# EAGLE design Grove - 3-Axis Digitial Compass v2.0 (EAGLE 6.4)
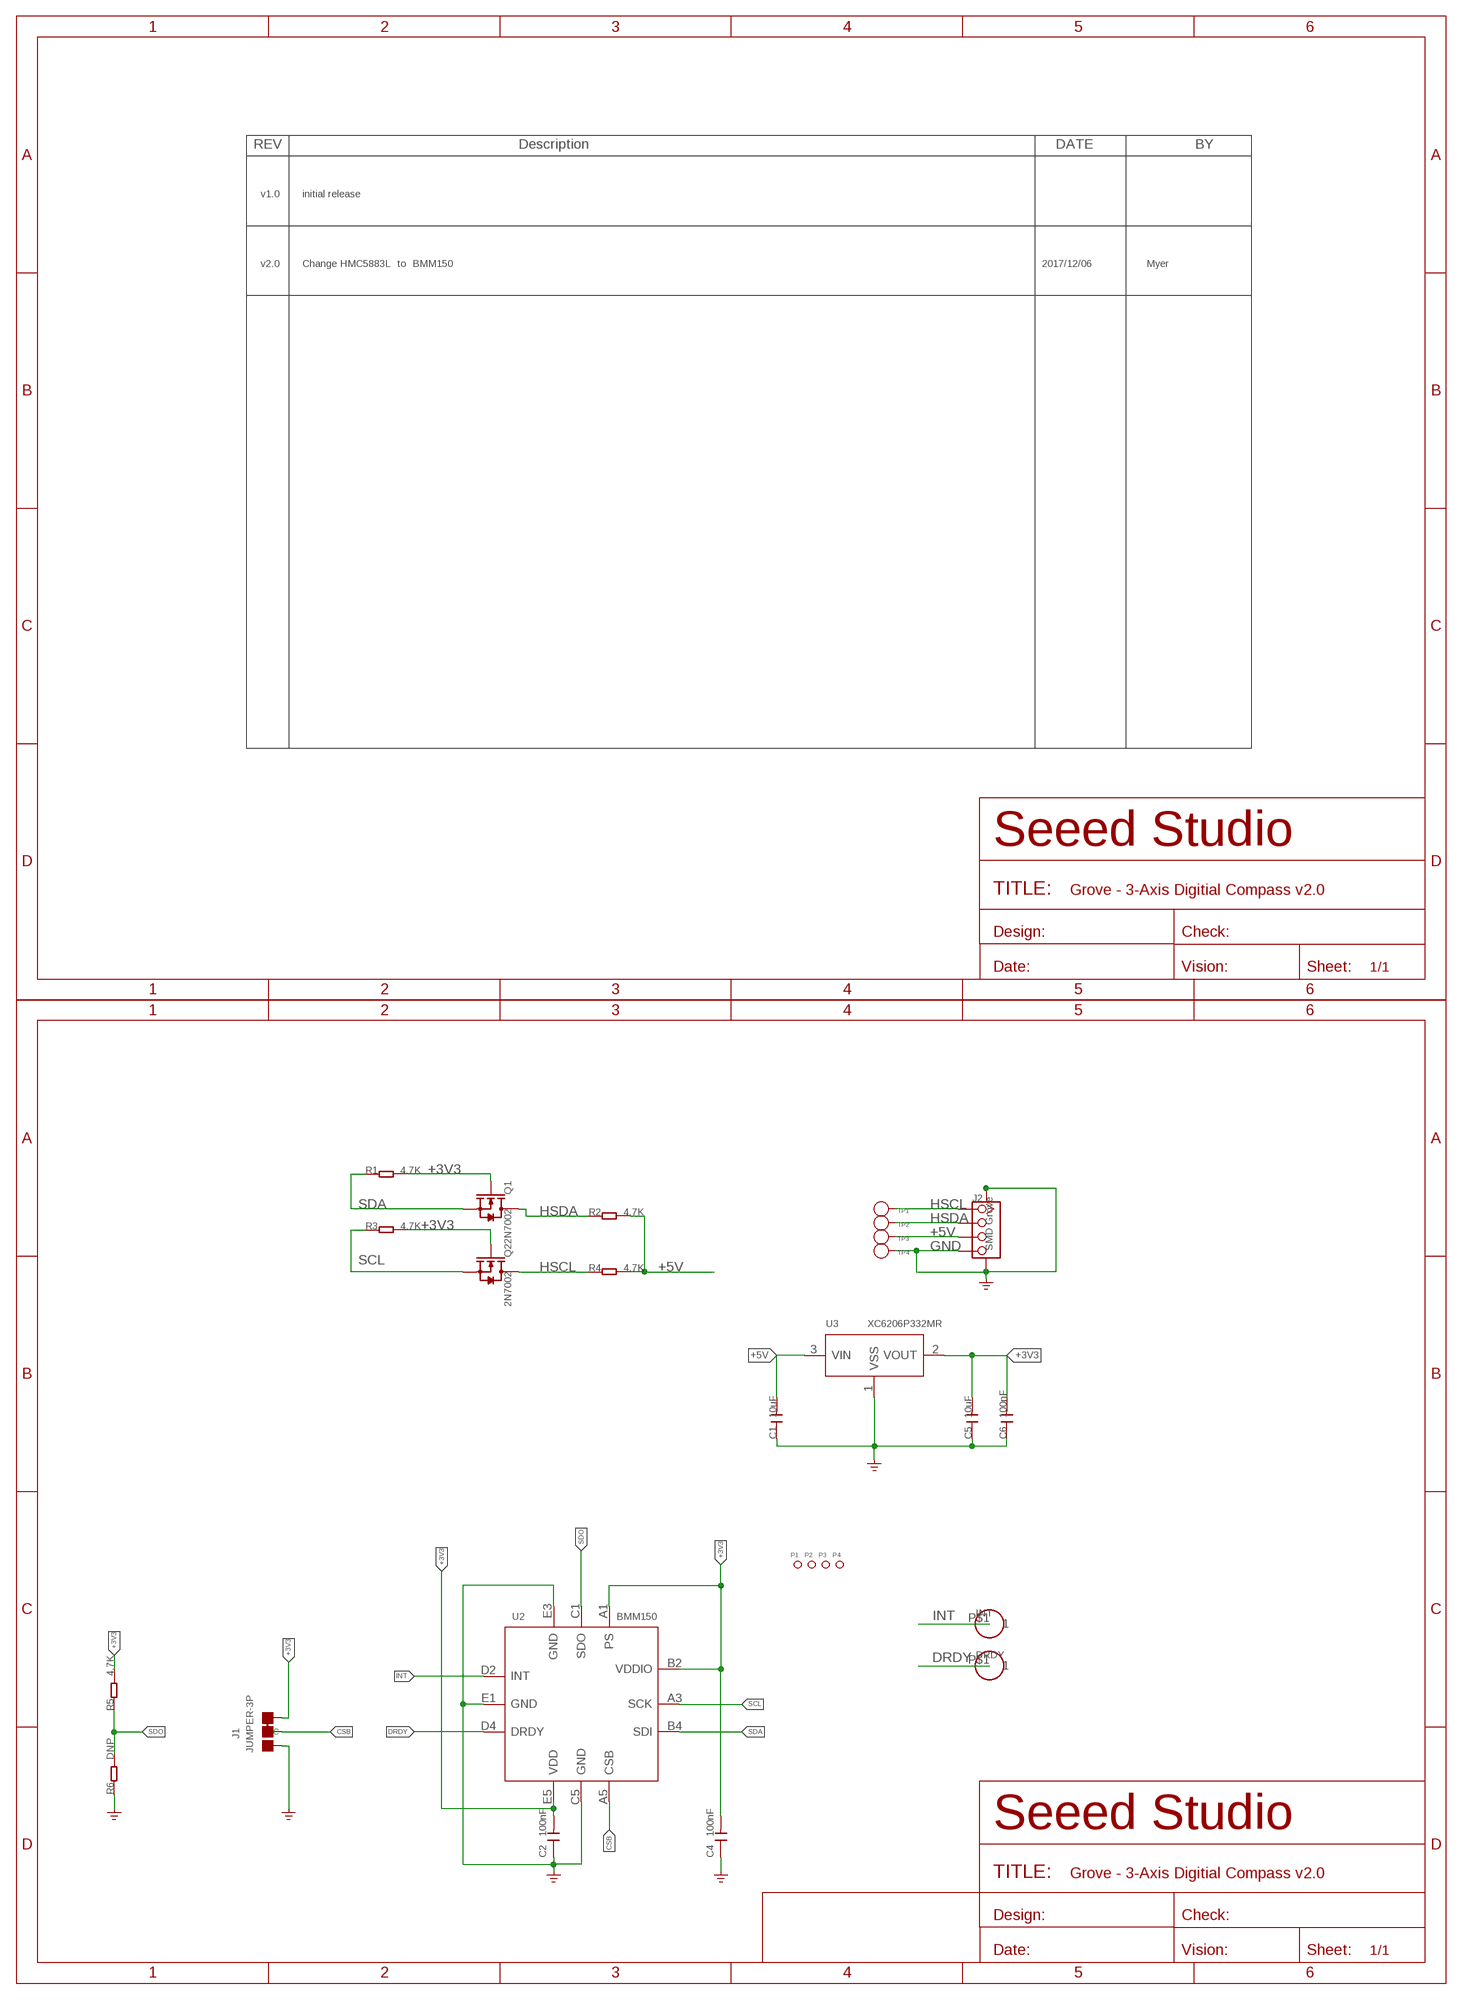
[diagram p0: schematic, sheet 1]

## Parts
C1  10uF  C-0603  [C0603]
C2  100nF  C-0603  [C0603]
C4  100nF  C-0603  [C0603]
C5  10uF  C-0603  [C0603]
C6  100nF  C-0603  [C0603]
DRDY  CK_1X132  [CK_1X1]
INT  CK_1X132  [CK_1X1]
J1  JUMPER-3P  JUMPER-3P-SHORT  [3P-SMD-SHORT]
J2  SMD Grove  TWIG-4P-2.0-SMD-FEMALE-REINFORCE'DD'  [4P-SMD-2.0]
P1  PAD-MARK'ANNULAR'  [ROUND-MARK-1.0]
P2  PAD-MARK'ANNULAR'  [ROUND-MARK-1.0]
P3  PAD-MARK'ANNULAR'  [ROUND-MARK-1.0]
P4  PAD-MARK'ANNULAR'  [ROUND-MARK-1.0]
Q1  2N7002  MOSFET-N'SOT23'  [SOT23]
Q2  2N7002  MOSFET-N'SOT23'  [SOT23]
R1  4.7K  R-0603  [R0603]
R2  4.7K  R-0603  [R0603]
R3  4.7K  R-0603  [R0603]
R4  4.7K  R-0603  [R0603]
R5  4.7K  R-0603  [R0603]
R6  DNP  R-0603  [R0603]
TP1  PAD-TEST-POINT'4545'  [TP_4545]
TP2  PAD-TEST-POINT'4545'  [TP_4545]
TP3  PAD-TEST-POINT'4545'  [TP_4545]
TP4  PAD-TEST-POINT'4545'  [TP_4545]
U2  BMM150  SENSOR-BMM150  [WLCS-1.56X1.56MM]
U3  XC6206P332MR  PMIC-XC6206PMR  [SOT-23]

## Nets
+3V3: C2.2 C4.2 C5.2 C6.2 J1.11(L) Q1.1(G) Q2.1(G) R1.2 R3.2 R5.2 U2.A1(PS) U2.B2(VDDIO) U2.E5(VDD) U3.2(VOUT)
+5V: C1.2 J2.3 R2.2 R4.2 TP3.T U3.3(VIN)
CSB: J1.MM(C) U2.A5(CSB)
DRDY: DRDY.P$1 U2.D4(DRDY)
GND: C1.1 C2.1 C4.1 C5.1 C6.1 J1.00(R) J2.4 J2.SS1 J2.SS2 R6.1 TP4.T U2.C5(GND) U2.E1(GND) U2.E3(GND) U3.1(VSS) ; supply symbol labelled GND_POWER
HSCL: J2.1 Q2.3(D) R4.1 TP1.T
HSDA: J2.2 Q1.3(D) R2.1 TP2.T
INT: INT.P$1 U2.D2(INT)
SCL: Q2.2(S) R3.1 U2.A3(SCK)
SDA: Q1.2(S) R1.1 U2.B4(SDI)
SDO: R5.1 R6.2 U2.C1(SDO)

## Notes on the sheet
- v1.0 | initial release
- v2.0 | Change HMC5883L  to  BMM150 | 2017/12/06 | Myer

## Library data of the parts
C1 C2 C4-C6 = Discrete:C*: Ceramic Capacitors
DRDY INT = CONNECTER1:CK_1X1
J1 = Discrete-new:JUMPER-3P-SHORT
J2 = Connector:TWIG-4P-2.0-SMD-FEMALE-REINFORCE
P1-P4 = Discrete:PAD-MARK; PARTNO: DNP
Q1 Q2 = Discrete:MOSFET-N: IRLL014: http://www.vishay.com/docs/91319/sihll014.pdf
R1-R6 = Discrete:R*
TP1-TP4 = Discrete:PAD-TEST-POINT; PARTNO: DNP
U2 = template:SENSOR-BMM150
U3 = IC-new:PMIC-XC6206P: LOW ESR Cap.Compatible Positive Voltage Regulators

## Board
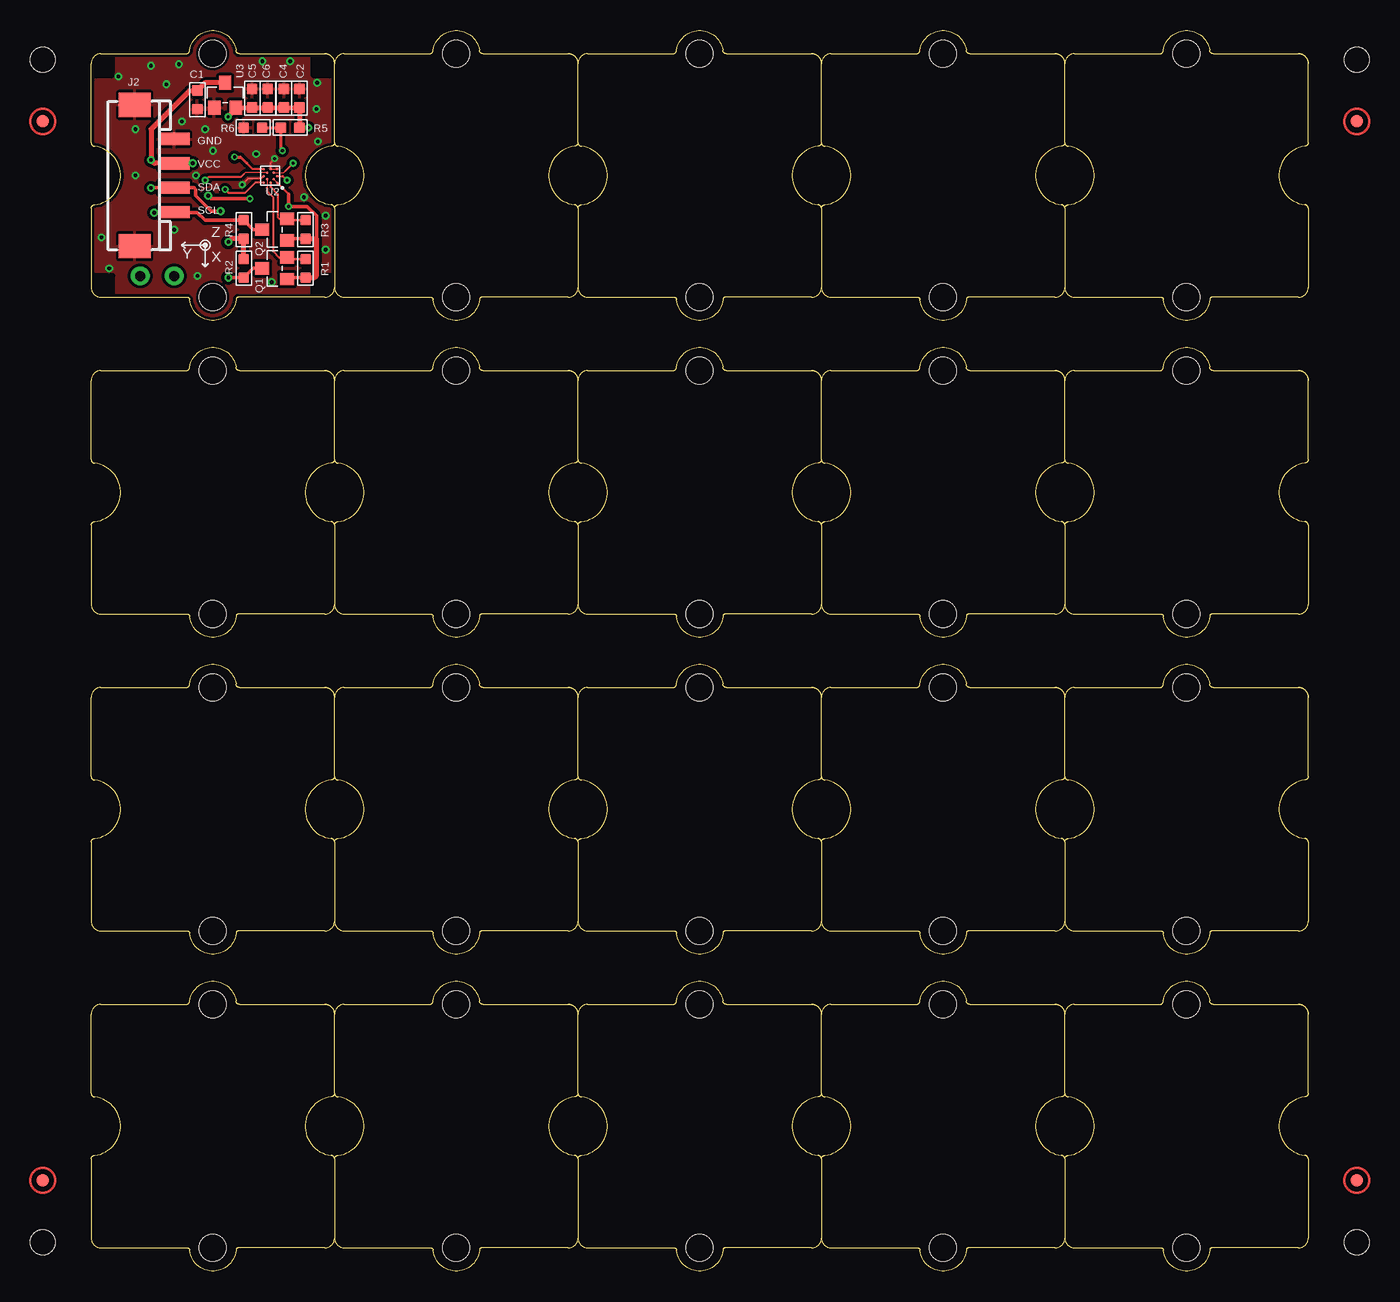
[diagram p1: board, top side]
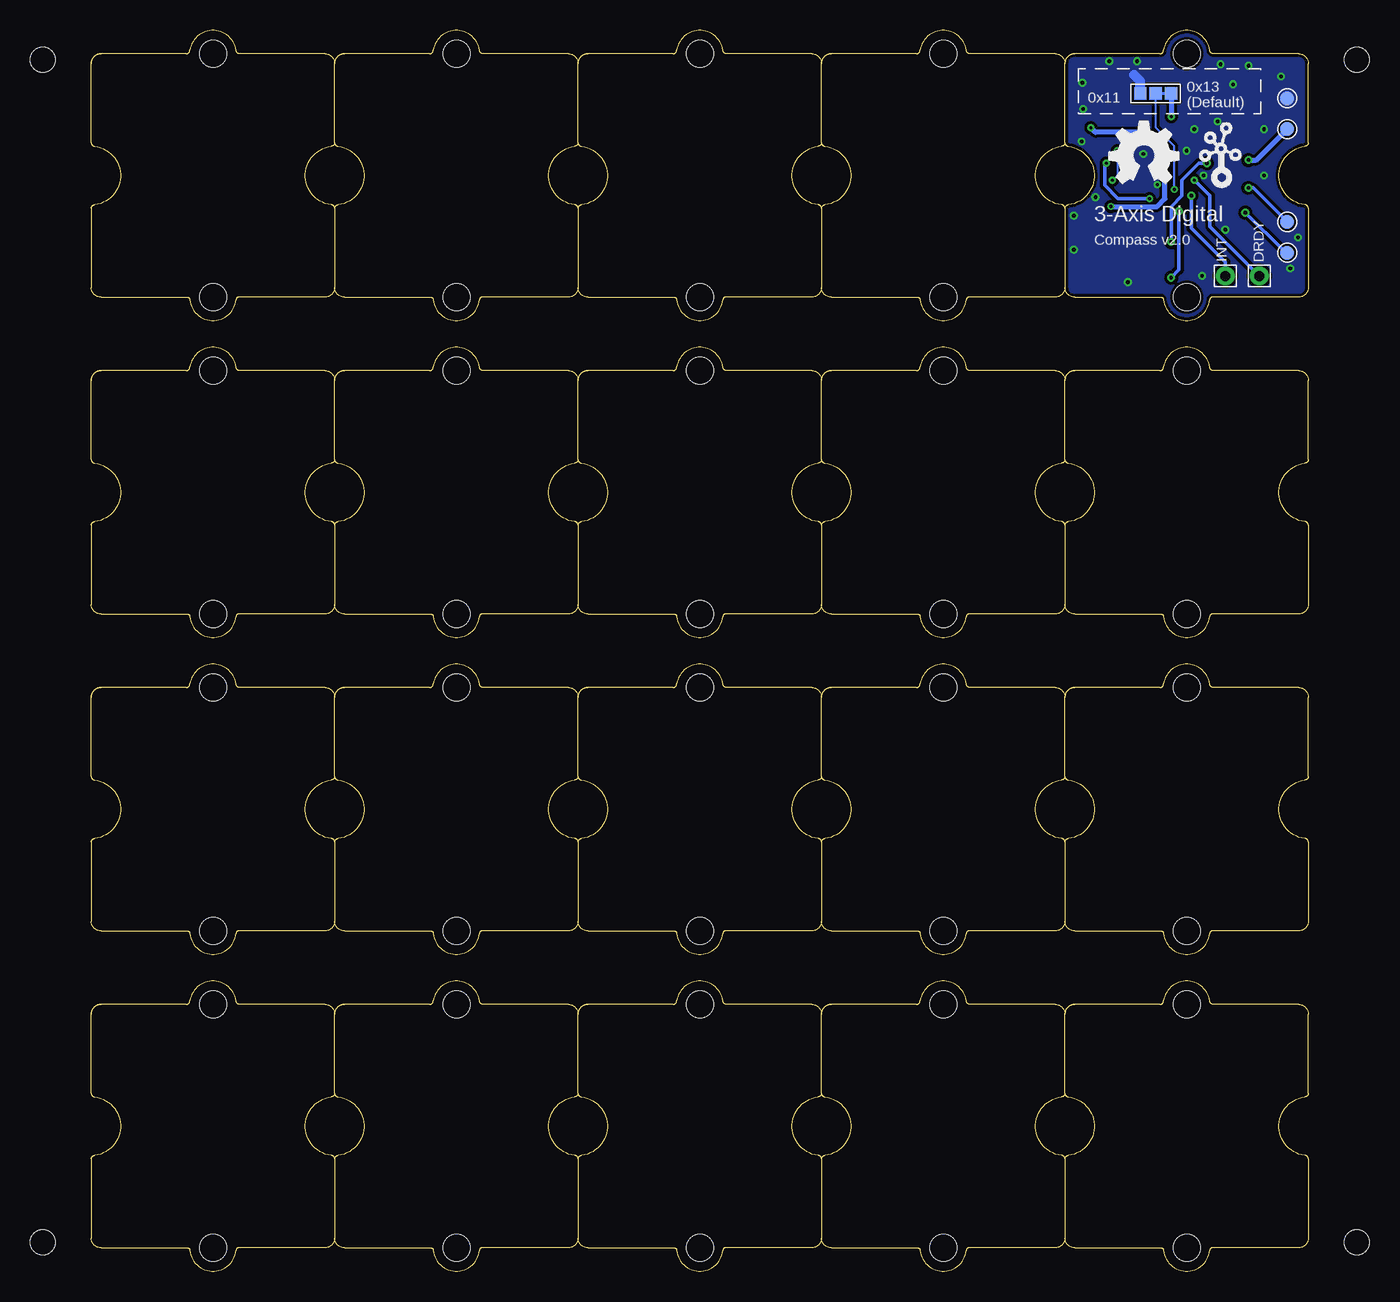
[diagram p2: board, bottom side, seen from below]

Size 100 x 101.93 mm. Coordinates in mm from the lower left corner, seen from the top.
Copper layers (1*16): Top 0.035mm / dielectric 1.5mm / Bottom 0.035mm
Design rules "SeeedStudio_2layer_DRU_no_angle_20140221 *": minimum track width 1mil, minimum drill 10mil, track to track 5mil, track to pad 5mil, pad to pad 5mil, via to via 5mil, smd to smd 0mil, copper to edge 10mil, drill to drill 10mil, minimum pad ring 10mil, minimum via ring 6mil, stop-mask expansion 2mil, vias tented up to drill 100mil, thermal gap 10mil
Holes 2.03 mm at -3.97,2.38 -3.97,99.54 103.98,99.54 103.98,2.38

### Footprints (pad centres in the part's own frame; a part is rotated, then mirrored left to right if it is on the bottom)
C0603 = smd 0.889 x 0.889: 1 -0.762,0; 2 0.762,0
CK_1X1 = drill 0.813 pad 1.524: P$1 0,0
3P-SMD-SHORT = smd 1.016 x 1.016: 00 -1.27,0; 11 1.27,0; MM 0,0
4P-SMD-2.0 = smd 1 x 2.54: 1 -3,0; 2 -1,0; 3 1,0; 4 3,0 | smd 2 x 2.6: SS1 -5.8,3.25; SS2 5.8,3.25
ROUND-MARK-1.0 = smd 1.016 x 1.016: P$1 0,0
SOT23 = smd 1.016 x 1.143: 1 -0.889,-1.016; 2 0.889,-1.016; 3 0,1.016
R0603 = smd 0.889 x 0.889: 1 -0.762,0; 2 0.762,0
TP_4545 = smd 1.143 x 1.143: T 0,0
WLCS-1.56X1.56MM = smd 0.2 x 0.2: A1 0.601,0.601; A3 0.601,0.035; A5 0.601,-0.531; B2 0.318,0.318; B4 0.318,-0.248; C1 0.035,0.601; C5 0.035,-0.531; D2 -0.248,0.318; D4 -0.248,-0.248; E1 -0.531,0.601; E3 -0.531,0.035; E5 -0.531,-0.531
SOT-23 = smd 1.016 x 1.143: 1 -0.889,-1.016; 2 0.889,-1.016; 3 0,1.016
1U-DIM-W/-DRILL = hole 2.2: 0,-10; 0,10

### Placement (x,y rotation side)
C1  8.73,96.24 90 top
C2  17.11,96.36 270 top
C4  15.84,96.36 270 top
C5  13.24,96.36 270 top
C6  14.51,96.36 270 top
DRDY  4.03,81.76 0 bottom
INT  6.83,81.76 270 bottom
J1  12.54,96.74 0 bottom
J2  6.83,90.01 90 top
P1  not placed on the board
P2  not placed on the board
P3  not placed on the board
P4  not placed on the board
Q1  15.08,82.39 90 top
Q2  15.08,85.57 90 top
R1  17.62,82.39 270 top
R2  12.54,82.39 90 top
R3  17.62,85.57 270 top
R4  12.54,85.57 270 top
R5  16.35,93.95 0 top
R6  13.3,93.95 0 top
TP1  1.74,83.66 0 bottom
TP2  1.74,86.2 0 bottom
TP3  1.74,93.82 0 bottom
TP4  1.74,96.36 0 bottom
U2  14.7,90.01 270 top
U3  11.02,96.62 0 top
U$3  [1U-DIM-W/-DRILL]  30,90.01 0 top
U$4  [1U-DIM-W/-DRILL]  10,90.01 0 top
U$8  [OSHW_FILLX200_NOTEXT]  16.35,89.38 0 bottom
U$9  [1U-DIM-W/-DRILL]  50,90.01 0 top
U$10  [1U-DIM-W/-DRILL]  70,90.01 0 top
U$11  [1U-DIM-W/-DRILL]  90,90.01 0 top
U$12  [1U-DIM-W/-DRILL]  10,63.98 0 top
U$13  [1U-DIM-W/-DRILL]  30,63.98 0 top
U$14  [1U-DIM-W/-DRILL]  50,63.98 0 top
U$15  [1U-DIM-W/-DRILL]  70,63.98 0 top
U$16  [1U-DIM-W/-DRILL]  90,63.98 0 top
U$17  [1U-DIM-W/-DRILL]  10,37.94 0 top
U$18  [1U-DIM-W/-DRILL]  30,37.94 0 top
U$19  [1U-DIM-W/-DRILL]  50,37.94 0 top
U$20  [1U-DIM-W/-DRILL]  70,37.94 0 top
U$21  [1U-DIM-W/-DRILL]  90,37.94 0 top
U$22  [1U-DIM-W/-DRILL]  10,11.91 0 top
U$23  [1U-DIM-W/-DRILL]  30,11.91 0 top
U$24  [1U-DIM-W/-DRILL]  50,11.91 0 top
U$25  [1U-DIM-W/-DRILL]  70,11.91 0 top
U$26  [1U-DIM-W/-DRILL]  90,11.91 0 top
U$31  [GROVE-SILK-SMALL]  9.37,88.87 0 bottom

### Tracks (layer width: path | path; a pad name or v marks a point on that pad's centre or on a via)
+3V3  (via drill 0.25 pad 0.51)
  Top 0.102: U2.B2 U2.A1
  Top 0.152: U2.E5 13.28,90.54 12.79,91.03 | U2.A1 16.22,88.49
  Top 0.254: v11.78,91.54 12.29,91.54 12.79,91.03
  Top 0.305: R1.2 16.22,81.63 Q1.1 | R3.2 16.1,84.81 Q2.1 | 12.92,95.28 C5.2 | 16.22,88.49 v16.22,87.47 17.75,87.47 18.51,86.71 18.51,84.3
  Top 0.406: R1.2 18.38,81.63 18.51,81.76 18.51,84.3 18.51,84.68 18.38,84.81 | R3.2 18.38,84.81 | 18.38,84.81 18.51,84.81 | v11.27,94.84 11.9,95.47 U3.2 C5.2 C6.2 C4.2 C2.2 R5.2 v17.87,93.95
  Bottom 0.406: v16.22,87.47 12.41,87.47 11.78,88.11 v11.78,91.54 11.78,92.05 13.3,93.57 17.49,93.57 v17.87,93.95 | J1.11 v11.27,94.84
+5V  (via drill 0.3 pad 0.64)
  Top 0.406: v8.35,91.03 6.97,91.03 6.95,91.01 | R2.2 R4.2 | R4.2 12.54,84.93 | J2.3 5.19,91.01 v4.92,91.28 4.92,93.82 8.1,97 C1.2 9.37,97.63 U3.3 | R4.2 11.52,84.81 v11.27,84.55
  Top 0.61: J2.3 6.95,91.01 7.08,91.01 7.1,91.03
  Bottom 0.305: v11.27,84.55 11.27,87.47 10.38,88.36 10.38,89.63 8.98,91.03 v8.35,91.03
  Bottom 0.406: v4.92,91.28 4.29,91.28 TP3.T
CSB  (via drill 0.25 pad 0.51)
  Top 0.152: v11.02,88.87 11.27,88.62 12.67,88.62 13.46,89.41 U2.A5
  Bottom 0.152: v11.02,88.87 11.02,92.43 12.54,93.95 J1.MM
DRDY  (via drill 0.25 pad 0.51)
  Top 0.102: U2.D4 12.66,90.26 12.54,90.14
  Top 0.152: 12.54,90.14 12.29,89.89 9.62,89.89 v9.37,89.63
  Bottom 0.305: DRDY.P$1 8.1,85.82 8.1,88.36 v9.37,89.63
GND  (via drill 0.25 pad 0.51, 0.3 pad 0.64)
  Top 0.102: U2.E3 U2.E1
  Top 0.152: U2.E3 14.73,91.06 v15.08,91.41 | U2.C5 14.16,89.98 13.94,89.76 12.92,89.76 v12.41,89.25
  Bottom 0.813: J1.00 13.81,97.76 14.32,98.27
  other vias: 18.64,92.81 16.35,99.41 2.25,98.14 0.86,84.93 9.37,93.82 14.06,99.41 7.21,99.16 4.92,99.03 6.83,85.57 8.73,81.76 6.19,97.51 3.65,93.82 3.65,90.01 1.49,82.39 19.27,86.71 19.27,83.92 17.49,88.24 10,92.05 8.6,90.01 14.83,81.25 13.56,91.79 7.46,94.46 18.51,95.47 18.57,97.63
  pour Top (isolate 0.254): -0.79,102.71 20.8,102.71 20.8,77.95 20.8,77.31 -0.79,77.31
  pour Bottom (isolate 0.254): -0.79,102.71 20.8,102.71 20.8,77.95 20.8,77.31 -0.79,77.31
HSCL  (via drill 0.3 pad 0.64)
  Top 0.305: Q2.3 13.3,85.57 R4.1 9.37,86.33 8.73,86.97 6.87,86.97 J2.1 5.22,87.01 v5.17,86.97
  Bottom 0.305: TP1.T 1.74,83.79 2,83.79 v5.17,86.97
HSDA  (via drill 0.3 pad 0.64)
  Top 0.305: v4.92,89 4.94,89.01 J2.2 6.84,89 8.48,89 8.6,88.87 8.6,88.36 9.87,87.09 v10.63,87.09 10.63,87.11 | Q1.3 13.3,82.39 R2.1 v11.27,81.63
  Bottom 0.305: v4.92,89 4.54,89 TP2.T | v11.27,81.63 10.63,82.27 v10.63,87.09
INT  (via drill 0.25 pad 0.51, 0.3 pad 0.64)
  Top 0.102: U2.D2 15.84,90.26 15.97,90.39
  Top 0.152: 15.97,90.39 v16.6,91.03
  Top 0.305: v13.05,88.11 9.87,88.11 v9.62,88.36
  Bottom 0.305: v13.05,88.11 15.64,88.11 16.73,89.2 16.73,90.9 v16.6,91.03 | INT.P$1 6.83,82.9 9.62,85.7 v9.62,88.36
SCL
  Top 0.152: U2.A3 14.73,89.09 15.33,88.49 15.33,86.58 15.46,86.46 Q2.2
  Top 0.203: R3.1 16.22,86.33 Q2.2 15.97,86.46 15.97,86.71 15.84,86.84
SDA
  Top 0.102: U2.B4 14.45,88.99
  Top 0.152: Q1.2 15.46,83.28 14.95,83.79 14.95,88.24 14.45,88.74 14.45,88.99
  Top 0.203: 15.97,83.28 Q1.2 16.22,83.16 R1.1
SDO  (via drill 0.25 pad 0.51)
  Top 0.152: U2.C1 15.75,89.98 v16.1,89.63
  Top 0.254: R6.2 R5.1 15.59,92.17 v15.71,92.05
  Bottom 0.152: v15.71,92.05 15.71,90.01 v16.1,89.63

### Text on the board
tPlace: GND | VCC | SDA | SCL | Z | Y | X
bPlace: 0x13 | (Default) | 0x11 | 3-Axis Digital | Compass v2.0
